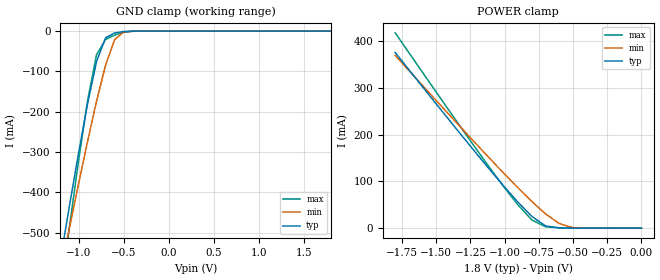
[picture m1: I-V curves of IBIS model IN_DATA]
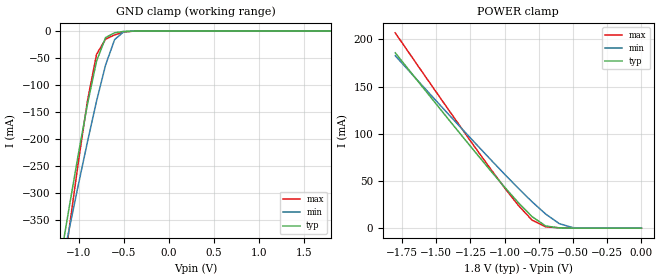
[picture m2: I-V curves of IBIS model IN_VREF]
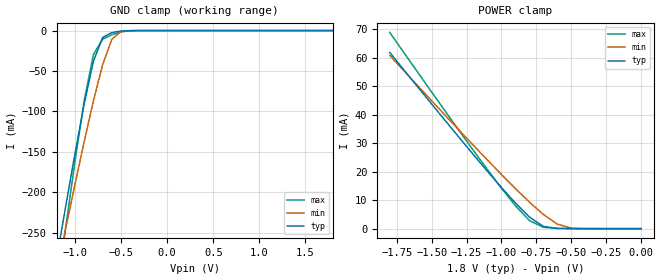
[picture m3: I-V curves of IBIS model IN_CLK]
| IBIS file 4pw865cy_t.ibs created by s2ibis2 version 1.2
| North Carolina State University Electronics Research Laboratory  1995
[IBIS ver]   2.1
[File name]   4pw865cy_t.ibs
[File Rev]   2.0
[Date]   Monday, July 12, 2004
[Source]   IDT
[Notes]   1. Temp typ=25C, min=0C, max=110C
   2. IDT C11.5 1.8V 1P 2-6M process
   3. Ramp rates based on 10Gig ohm load
[Disclaimer]
READ THESE TERMS AND CONDITIONS CAREFULLY BEFORE USING THIS IBIS MODEL.  BY
USING THIS IBIS MODEL, YOU ARE ACCEPTING AND AGREEING TO THESE TERMS AND
CONDITIONS OF USE.
Integrated Device Technology, Inc. ("IDT") hereby grants the user of this
IBIS model ("User") a non-exclusive, nontransferable license to use this
IBIS model under the following terms: The User is granted this license only
to use the IBIS model for demonstration purposes only and is not granted
rights to sell, copy (except as needed to run the IBIS model), rent, lease
or sub-license (except for demonstration) the IBIS model in whole or in
part, or in modified form to anyone. The User may modify the IBIS model to
suit its specific applications, but  rights to derivative works and such
modifications shall belong to IDT.
THIS IBIS MODEL IS PROVIDED ON AN AS IS" BASIS AND IDT  MAKES ABSOLUTELY NO
WARRANTY WITH RESPECT TO THE INFORMATION CONTAINED HEREIN.  IDT DISCLAIMS
AND USER WAIVES ALL WARRANTIES, EXPRESS AND IMPLIED, INCLUDING WARRANTIES OF
MERCHANTABILITY AND FITNESS FOR A PARTICULAR PURPOSE.  THE ENTIRE RISK AS TO
QUALITY AND PERFORMANCE IS WITH THE USER  ACCORDINGLY, IN NO EVENT SHALL IDT
BE LIABLE FOR ANY DIRECT OR INDIRECT DAMAGES, WHETHER IN CONTRACT OR TORT,
INCLUDING ANY LOST PROFITS OR OTHER INCIDENTAL, CONSEQUENTIAL, EXEMPLARY, OR
PUNITIVE DAMAGES ARISING OUT OF THE USE OR APPLICATION OF THE  IBIS MODEL,
WHETHER OR NOT IDT HAD NOTICE OF SUCH DAMAGES.
IDT reserves the right to make changes without notice to any product herein
to improve reliability, function, or design. IDT does not convey any license
under patent rights or any other intellectual property rights, including
those of third parties. IDT is not obligated to provide  maintenance or
support for the licensed IBIS model.
This model is for the 28 bit 1:2 Registered Buffer With Parity
[Copyright]
Copyright 2002, Integrated Device Technology, Inc. All rights
reserved.
|   Component IDT4PW865CY
[Component]   IDT4PW865CY
[Manufacturer]   Integrated Device Technology, Inc.
[Package]
|Following package RLC parasitics are for the 160 pin TFBGA package
| variable   typ   min   max
R_pkg   0.17200   0.17200   0.17200
L_pkg   3.38000nH   3.38000nH   3.38000nH
C_pkg   0.74300pF   0.74300pF   0.74300pF
[Pin]  signal_name   model_name   R_pin   L_pin   C_pin
A1   VREF   IN_VREF
A2   NC   NC
A3   PARIN   IN_PARIN
A4   NC   NC
A5   NC   NC
A6   QCKE1A   OUTBUF
A7   QCKE0A   OUTBUF
A8   Q21A   OUTBUF
A9   Q19A   OUTBUF
A10   Q18A   OUTBUF
A11   Q17B   OUTBUF
A12   Q17A   OUTBUF
B1   D1   IN_DATA
B2   D2   IN_DATA
B3   NC   NC
B4   NC   NC
B5   NC   NC
B6   QCKE1B   OUTBUF
B7   QCKE0B   OUTBUF
B8   Q21B   OUTBUF
B9   Q19B   OUTBUF
B10   Q18B   OUTBUF
B11   QODT0B   OUTBUF
B12   QODT0A   OUTBUF
C1   D3   IN_DATA
C2   D4   IN_DATA
C3   NC   NC
C4   NC   NC
C5   NC   NC
C6   NC   NC
C7   NC   NC
C8   NC   NC
C9   NC   NC
C10   NC   NC
C11   QODT1B   OUTBUF
C12   QODT1A   OUTBUF
D1   D6   IN_DATA
D2   D5   IN_DATA
D3   NC   NC
D4   VDDL   POWER
D5   GND   GND
D6   NC   NC
D7   NC   NC
D8   GND   GND
D9   GND   GND
D10   NC   NC
D11   Q20B   OUTBUF
D12   Q20A   OUTBUF
E1   D7   IN_DATA
E2   D8   IN_DATA
E3   NC   NC
E4   VDDL   POWER
E5   GND   GND
E6   VDDL   POWER
E7   VDDR   POWER
E8   GND   GND
E9   GND   GND
E10   NC   NC
E11   Q16B   OUTBUF
E12   Q16A   OUTBUF
F1   D11   IN_DATA
F2   D9   IN_DATA
F3   NC   NC
F4   VDDL   POWER
F5   GND   GND
F6   NC   NC
F7   NC   NC
F8   VDDR   POWER
F9   VDDR   POWER
F10   NC   NC
F11   Q1B   OUTBUF
F12   Q1A   OUTBUF
G1   D18   IN_DATA
G2   D12   IN_DATA
G3   NC   NC
G4   VDDL   POWER
G5   GND   GND
G6   NC   NC
G7   NC   NC
G8   VDDR   POWER
G9   VDDR   POWER
G10   NC   NC
G11   Q2B   OUTBUF
G12   Q2A   OUTBUF
H1   CSGATEEN   IN_CSGATEN
H2   D15   IN_DATA
H3   NC   NC
H4   VDDL   POWER
H5   GND   GND
H6   NC   NC
H7   NC   NC
H8   GND   GND
H9   GND   GND
H10   NC   NC
H11   Q5B   OUTBUF
H12   Q5A   OUTBUF
J1   CLK   IN_CLK
J2   _DCS0_   IN_DATA
J3   NC   NC
J4   GND   GND
J5   GND   GND
J6   NC   NC
J7   NC   NC
J8   VDDR   POWER
J9   VDDR   POWER
J10   NC   NC
J11   _QCS0B_   OUTBUF
J12   _QCS0A_   OUTBUF
K1   _CLK_   IN_CLK
K2   _DCS1_   IN_DATA
K3   NC   NC
K4   VDDL   POWER
K5   VDDL   POWER
K6   NC   NC
K7   NC   NC
K8   GND   GND
K9   GND   GND
K10   NC   NC
K11   _QCS1B_   OUTBUF
K12   _QCS1A_   OUTBUF
L1   _RESET_   IN_RESET
L2   D14   IN_DATA
L3   NC   NC
L4   GND   GND
L5   GND   GND
L6   NC   NC
L7   NC   NC
L8   VDDR   POWER
L9   VDDR   POWER
L10   NC   NC
L11   Q6B   OUTBUF
L12   Q6A   OUTBUF
M1   D0   IN_DATA
M2   D10   IN_DATA
M3   NC   NC
M4   GND   GND
M5   GND   GND
M6   NC   NC
M7   NC   NC
M8   GND   GND
M9   GND   GND
M10   NC   NC
M11   Q10B   OUTBUF
M12   Q10A   OUTBUF
N1   D17   IN_DATA
N2   D16   IN_DATA
N3   NC   NC
N4   VDDL   POWER
N5   VDDL   POWER
N6   NC   NC
N7   NC   NC
N8   VDDR   POWER
N9   VDDR   POWER
N10   NC   NC
N11   Q9B   OUTBUF
N12   Q9A   OUTBUF
P1   D19   IN_DATA
P2   D21   IN_DATA
P3   NC   NC
P4   GND   GND
P5   VDDL   POWER
P6   VDDL   POWER
P7   VDDR   POWER
P8   VDDR   POWER
P9   GND   GND
P10   NC   NC
P11   Q11B   OUTBUF
P12   Q11A   OUTBUF
R1   D13   IN_DATA
R2   D20   IN_DATA
R3   NC   NC
R4   GND   GND
R5   VDDL   POWER
R6   VDDL   POWER
R7   GND   GND
R8   GND   GND
R9   GND   GND
R10   NC   NC
R11   Q15B   OUTBUF
R12   Q15A   OUTBUF
T1   DODT1   IN_DATA
T2   DODT0   IN_DATA
T3   NC   NC
T4   NC   NC
T5   NC   NC
T6   NC   NC
T7   NC   NC
T8   NC   NC
T9   NC   NC
T10   NC   NC
T11   Q14B   OUTBUF
T12   Q14A   OUTBUF
U1   DCKE0   IN_DATA
U2   DCKE1   IN_DATA
U3   MCL/GND   GND
U4   _PTYERR_   OUT_PTYERR
U5   MCH/VDDL   POWER
U6   Q3B   OUTBUF
U7   Q12B   OUTBUF
U8   Q7B   OUTBUF
U9   Q4B   OUTBUF
U10   Q13B   OUTBUF
U11   Q0B   OUTBUF
U12   Q8B   OUTBUF
V1   VREF   IN_VREF
V2   MCL/GND   GND
V3   MCL/GND   GND
V4   NC   NC
V5   MCH/VDDL   POWER
V6   Q3A   OUTBUF
V7   Q12A   OUTBUF
V8   Q7A   OUTBUF
V9   Q4A   OUTBUF
V10   Q13A   OUTBUF
V11   Q0A   OUTBUF
V12   Q8A   OUTBUF
| din  din   dummy_model
| err  err   dummy_model
[Diff Pin]  inv_pin   vdiff   tdelay_typ  tdelay_min  tdelay_max
J1   K1   0.60000V  NA   |CLK<P:N> Input  Pair
| Models and submodels in the file (8): IN_DATA (Input), IN_VREF (Input), IN_CLK (Input), IN_CSGATEN (Input), IN_PARIN (Input), IN_RESET (Input), OUT_PTYERR (Open_sink), OUTBUF (Output)
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|   Model IN_DATA
[Model]   IN_DATA
Model_type   Input
Vinl =  0.65000V
Vinh =  1.15000V
C_comp   3.00000pF   3.0000pF   3.00000pF
[Temperature Range]   25.00000   0.11000k   0.000
[Voltage Range]   1.80000V   1.70000V   1.90000V
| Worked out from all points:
|   GND clamp passes 1 mA (typ) near -0.50 V on its own axis
|   POWER clamp passes 1 mA (typ) near -0.61 V on its own axis
[GND_clamp]
| voltage   I(typ)   I(min)   I(max)
-1.8V     -1.389A    -1.277A    -1.696A
-1.2V     -565.6mA   -597.8mA   -652.3mA
-1.1V     -432.8mA   -487.6mA   -484.7mA
-1V       -303.5mA   -379.2mA   -322.7mA
-900mV    -180.9mA   -273.9mA   -172.6mA
-800mV    -75.06mA   -173.7mA   -58.49mA
-700mV    -16.66mA   -84.24mA   -20.86mA
-600mV    -4.62mA    -21.4mA    -9.97mA
-500mV    -1.021mA   -2.066mA   -3.095mA
-300mV    -22.94uA   -31.32uA   -73.59uA
1.8V      25.83nA    16.72nA    180.9nA
[POWER_clamp]
| voltage   I(typ)   I(min)   I(max)
-1.8V     375.1mA    369.1mA    417.2mA
-1.4V     229mA      240.6mA    248.6mA
-1.1V     122mA      146.1mA    125.4mA
-900mV    54.54mA    85.39mA    48.68mA
-800mV    24.76mA    56.61mA    17.27mA
-700mV    4.694mA    30.23mA    2.901mA
-600mV    379.5uA    9.628mA    728.6uA
-500mV    44.96uA    1.062mA    142.5uA
0V        583.5pA    1.142nA    186.4nA
|   Model IN_VREF
[Model]   IN_VREF
Model_type   Input
Vinl =  0.83300V
Vinh =  0.96900V
C_comp   3.00000pF   3.0000pF   3.00000pF
[Temperature Range]   25.00000   0.11000k   0.000
[Voltage Range]   1.80000V   1.70000V   1.90000V
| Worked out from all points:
|   GND clamp passes 1 mA (typ) near -0.52 V on its own axis
|   POWER clamp passes 1 mA (typ) near -0.64 V on its own axis
[GND_clamp]
| voltage   I(typ)   I(min)   I(max)
-1.8V     -1.039A    -955.2mA   -1.269A
-1.2V     -422.7mA   -446.9mA   -487.6mA
-1.1V     -323.3mA   -364.4mA   -362.1mA
-1V       -226.5mA   -283.4mA   -240.8mA
-900mV    -134.8mA   -204.6mA   -128.4mA
-800mV    -55.62mA   -129.6mA   -43.04mA
-700mV    -12mA      -62.76mA   -15.01mA
-600mV    -3.135mA   -15.78mA   -7.026mA
-500mV    -579.5uA   -1.401mA   -2.034mA
-300mV    -1.767uA   -3.73uA    -8.578uA
1.8V      17.76pA    8.181nA    -22.5pA
[POWER_clamp]
| voltage   I(typ)   I(min)   I(max)
-1.8V     185.8mA    182.7mA    206.9mA
-1.4V     113.4mA    119mA      123.3mA
-1.1V     60.42mA    72.28mA    62.15mA
-900mV    26.99mA    42.23mA    24.11mA
-800mV    12.24mA    27.99mA    8.537mA
-700mV    2.309mA    14.93mA    1.433mA
-600mV    187.3uA    4.737mA    363.9uA
-500mV    22.39uA    519.1uA    71.04uA
0V        17.76pA    571.4pA    5.824pA
|   Model IN_CLK
[Model]   IN_CLK
Model_type   Input
Vinl =  0.37500V
Vinh =  1.42500V
C_comp   5.00000pF   5.0000pF   5.00000pF
[Temperature Range]   25.00000   0.11000k   0.000
[Voltage Range]   1.80000V   1.70000V   1.90000V
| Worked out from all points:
|   GND clamp passes 1 mA (typ) near -0.52 V on its own axis
|   POWER clamp passes 1 mA (typ) near -0.71 V on its own axis
[GND_clamp]
| voltage   I(typ)   I(min)   I(max)
-1.8V     -696.8mA   -640.7mA   -850.1mA
-1.2V     -283.6mA   -299.9mA   -327.1mA
-1.1V     -217.1mA   -244.6mA   -243.2mA
-1V       -152.3mA   -190.3mA   -162mA
-900mV    -90.9mA    -137.4mA   -86.86mA
-800mV    -37.86mA   -87.16mA   -29.67mA
-700mV    -8.545mA   -42.31mA   -10.73mA
-600mV    -2.425mA   -10.78mA   -5.167mA
-500mV    -549.6uA   -1.041mA   -1.631mA
-300mV    -6.609uA   -5.177uA   -26.84uA
1.8V      493.5pA    3.208nA    373.7pA
[POWER_clamp]
| voltage   I(typ)   I(min)   I(max)
-1.8V     61.94mA    60.89mA    68.97mA
-1.4V     37.81mA    39.68mA    41.1mA
-1.1V     20.14mA    24.09mA    20.72mA
-900mV    8.997mA    14.08mA    8.037mA
-800mV    4.08mA     9.329mA    2.846mA
-700mV    769.7uA    4.978mA    477.8uA
-600mV    62.43uA    1.581mA    121.3uA
-500mV    7.465uA    173uA      23.68uA
0V        493.5pA    646.3pA    416.8pA
